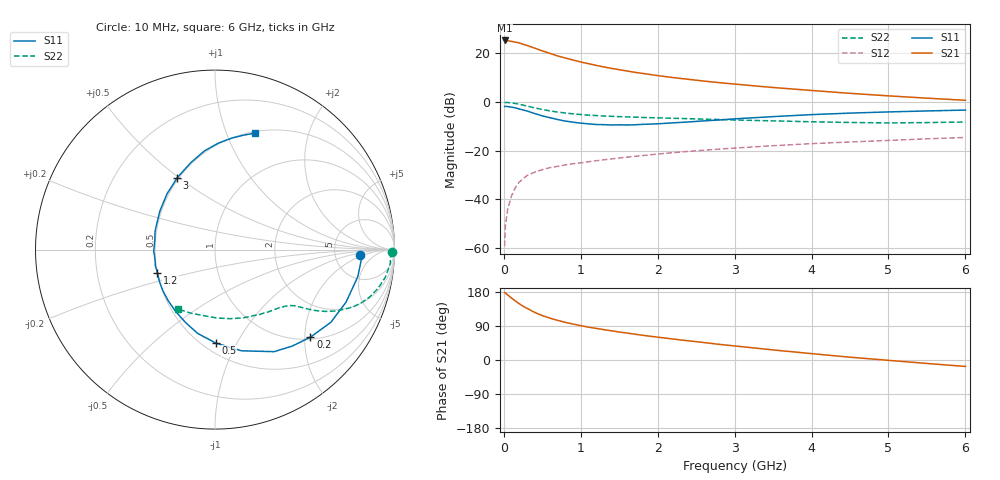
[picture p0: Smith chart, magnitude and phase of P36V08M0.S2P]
! SIEMENS Small Signal Semiconductors
! BFP181
! Si NPN RF Bipolar Junction Transistor in SOT143
! VCE = 6 V  IC = 8 mA
! Common Emitter S-Parameters:  March  1996
# GHz  S  MA  R  50
!  f  S11  S21  S12  S22
! GHz  MAG  ANG  MAG  ANG  MAG  ANG  MAG  ANG
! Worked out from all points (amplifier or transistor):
!   36 points, 10 MHz to 6 GHz, reference 50 ohm
!   highest |S21| = 25.3 dB at 10 MHz (marker M1)
!   |S21| within 3 dB of that: start of sweep to 387.1 MHz
!   unconditionally stable (mu >= 1): 1.439 GHz to end of sweep
!   at 250 MHz: K = 0.28, MSG = 27.6 dB, |S12| = -31.5 dB
!   at 1.4 GHz: K = 0.99, MSG = 18.6 dB, |S12| = -23.3 dB
!   at 6 GHz: K = 1.03, MAG = 6.5 dB, |S12| = -14.5 dB
!   S11 on the Smith chart (normalised r, x): 10 MHz: 9.21, -1.58; 200 MHz: 1.05, -2.14; 500 MHz: 0.58, -0.83; 1.2 GHz: 0.50, -0.15; 3 GHz: 0.49, +0.49; 6 GHz: 0.52, +1.26
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0.01  0.8093 -2.1  18.41 177.7  0.0011 91.8  0.9851 -0.8
0.02  0.8166 -4.3  18.23 176.7  0.0029 91.1  0.9798 -1.8
0.05  0.8098 -10.7  18.2 171.5  0.0063 85.5  0.9795 -4.7
0.1  0.7868 -21.8  17.62 163.5  0.0119 77.7  0.9616 -9.2
0.15  0.762 -32.1  17.04 155.8  0.0175 73.5  0.9345 -13.3
0.2  0.7216 -42.5  16.4 148.5  0.0228 68.8  0.9017 -17.0
0.25  0.689 -51.2  15.39 141.9  0.0265 65.0  0.8642 -20.3
0.3  0.6573 -59.9  14.54 136.6  0.0309 61.5  0.8291 -22.8
0.4  0.5829 -75.3  12.82 125.7  0.0363 57.0  0.7609 -26.7
0.5  0.5206 -89.5  11.24 117.2  0.041 53.0  0.7035 -29.3
0.6  0.4771 -101.6  10.01 110.4  0.0451 50.5  0.6588 -31.1
0.7  0.438 -112.1  8.851 104.6  0.0479 49.2  0.6233 -32.3
0.8  0.4069 -123.0  8.032 99.3  0.0513 48.0  0.5957 -33.2
1.1  0.3568 -150.2  6.145 86.6  0.0596 46.4  0.5397 -35.4
1.2  0.3462 -157.9  5.67 83.4  0.0625 45.9  0.5285 -36.2
1.7  0.3411 168.9  4.093 68.2  0.077 44.9  0.4906 -40.9
2.2  0.3742 145.3  3.184 55.3  0.0914 43.1  0.4648 -46.9
3  0.4525 117.8  2.341 37.1  0.1136 38.5  0.4281 -58.9
3.5  0.5025 105.6  1.991 26.6  0.1271 35.0  0.4112 -67.8
4.5  0.5935 88.2  1.512 7.4  0.1515 27.5  0.3809 -88.7
5.5  0.6572 76.0  1.203 -9.1  0.176 20.9  0.3791 -110.8
6  0.6854 71.1  1.088 -17.0  0.1877 17.0  0.3902 -122.2
